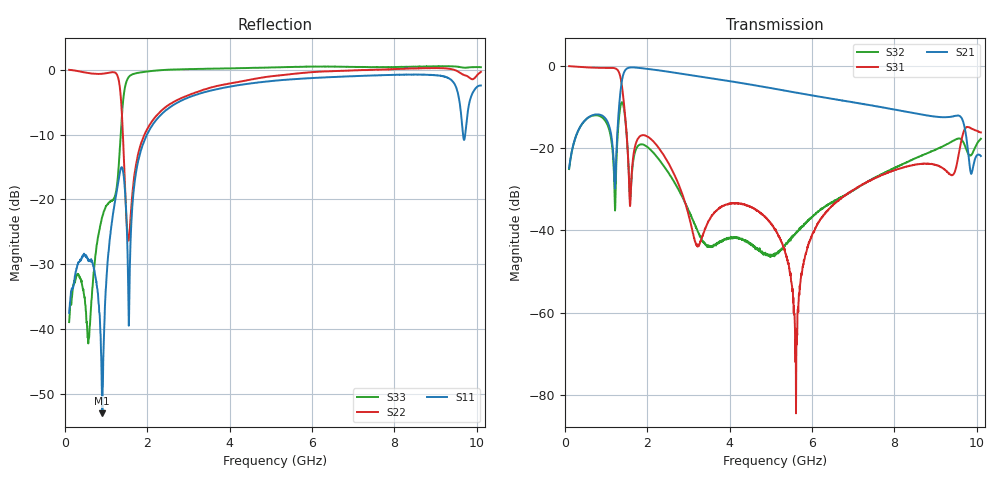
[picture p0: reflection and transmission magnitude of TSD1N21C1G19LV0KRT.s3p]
# MHZ S RI R 50
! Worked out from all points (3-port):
!   2001 points, 100 MHz to 10.1 GHz, reference 50 ohm
!   strongest paths, dB at 100 MHz, 2.6 GHz, 5.1 GHz, 7.6 GHz, 10.1 GHz:
!     S21: -24.9, -1.6, -5.6, -9.9, -21.9
!     S31: -0.1, -25.3, -39.6, -27.0, -16.2
!     S32: -25.1, -27.4, -46.0, -26.8, -17.7
!   lowest |S11| = -53.0 dB at 905 MHz (marker M1), VSWR 1.00, Z = 49.9 + j0.215 ohm
!   |S11| at or under -10 dB: start of sweep to 1.992 GHz; 9.667 GHz to 9.72 GHz (52.99 MHz wide, 0.547 % of centre)
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100  0.00584 -0.012  0.00847 0.056  0.9847 -0.1381
     0.00843 0.056  0.9607 -0.271  0.0154 0.0537
     0.9829 -0.1378  0.0154 0.0535  -0.0014 -0.0112
905  -0.000617 0.00215  0.2087 0.1332  0.2195 -0.9201
     0.2092 0.1338  -0.4277 -0.8269  0.1679 -0.1659
     0.2207 -0.92  0.1676 -0.1657  0.0731 -0.00435
1210  0.0849 -0.0428  0.012 0.0317  -0.5572 -0.7516
      0.0121 0.0318  -0.9184 -0.2526  0.00812 -0.019
      -0.5569 -0.7526  0.00824 -0.0189  0.0618 -0.0853
1360  0.0666 -0.162  -0.383 0.3974  -0.674 0.0344
      -0.3837 0.3972  -0.4148 0.4143  0.2692 -0.2164
      -0.6738 0.0344  0.2691 -0.2167  -0.3473 -0.0439
1715  0.1533 -0.012  0.6318 0.7184  -0.00857 -0.1116
      0.6308 0.7157  0.0031 -0.1774  0.0618 -0.0708
      -0.00839 -0.1115  0.0621 -0.0712  0.9351 -0.0803
3215  -0.1089 -0.6367  0.7331 -0.1804  0.000171 -0.00651
      0.7277 -0.1813  -0.2188 -0.6376  -0.00968 0.00256
      0.000245 -0.00645  -0.00955 0.00279  -0.2406 -0.9852
5100  -0.5997 -0.5629  0.3892 -0.3522  0.00767 -0.00683
      0.3896 -0.353  -0.5522 -0.7055  1.03e-06 0.00524
      0.00775 -0.00698  0.000132 0.00503  -0.7086 -0.7666
5615  -0.6996 -0.4786  0.3248 -0.3433  0.000339 0.000358
      0.3226 -0.3457  -0.5925 -0.7209  -0.00566 0.00752
      0.000116 0.000185  -0.00564 0.00732  -0.7271 -0.7618
6380  -0.8103 -0.3295  0.2434 -0.3257  -0.0099 0.0146
      0.2456 -0.3232  -0.6144 -0.7522  -0.0154 0.0138
      -0.0099 0.0145  -0.0155 0.0135  -0.7311 -0.7652
10100  -0.7523 0.0709  0.043 -0.0676  -0.0651 0.141
       0.0425 -0.0679  -0.8076 -0.5233  -0.0516 0.1192
       -0.064 0.1414  -0.0514 0.1193  -0.9948 -0.3216
